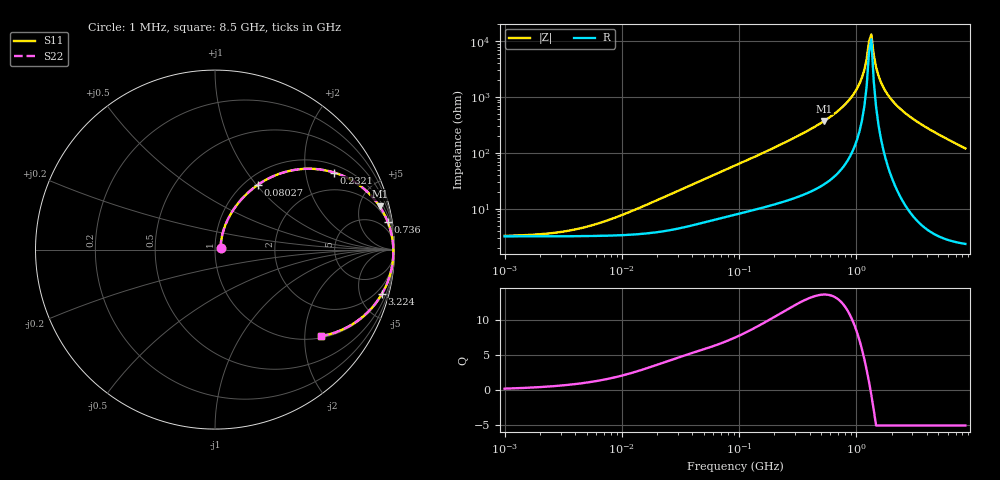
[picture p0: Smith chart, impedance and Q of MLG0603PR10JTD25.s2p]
! S-Parameter Data Generated by TDK Corporation
! Copyright(C) 2025 TDK Corporation.
! All Rights Reserved.
! TDK P/N: MLG0603PR10JTD25 (SMD / SMT Inductor (Coil))
! Property: L=100nH at 300MHz
! Size(LxWxT): 0.6x0.3x0.3mm
! Model Type: s2p (Touchstone File Format Version 1.0)
! Frequency: DC=Yes Start=1MHz Stop=8500MHz 198points Log-sweep
! Model Generated on Feb. 6, 2025
! Terms and conditions regarding TDK Simulation Models:
! 1)This simulation model is being provided solely for informational
!  purposes. Please refer to the specifications of the products in
!  terms of detailed characteristics of such products.
! 2)In no event shall TDK Corporation of any of its subsidiaries be
!  liable for any loss or damage arising, directly or indirectly,
!  from any information contained in this simulation model, including,
!  but not limited to loss or damages arising from any inaccuracies,
!  omissions or errors in connection with such information.
! 3)Any and all copyrights on this simulation model are owned by
!  TDK Corporation.  Duplication or redistribution of this simulation
!  model without prior written permission from TDK Corporation
!  is prohibited.
! 4)This simulation model is subject to any modification or change
!  without any prior notice.
! 5)Neither TDK Corporation nor any of its subsidiaries shall make any
!  warranty, express or implied, including but not limited to the
!  correctness, implied warranties of merchantability and fitness for
!  a particular purpose with respect to this simulation models.
! 6)The use of this simulation model shall be deemed to have consented
!  to the terms and conditions hereof.
! Port Assignments:
!  1 ---@@@--- 2
! Applicable Conditions:
!  Temperature = 25 degC
!  DC Bias Current = 0 A
!  Small Signal Operation
# Hz S MA R 50
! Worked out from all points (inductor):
!   197 points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, 1 MHz to 8.5 GHz, reference 50 ohm
!   read as one part in series: L = 109 nH near 15.95 MHz
!   highest Q = 13.5 at 532.8 MHz (marker M1), where L = 111 nH
!   self-resonance near 1.281 GHz
!   S11 on the Smith chart (normalised r, x): 1 MHz: 1.06, +0.01; 80.27 MHz: 1.15, +1.02; 232.1 MHz: 1.26, +2.88; 736 MHz: 2, +12; 3.224 GHz: 1.13, -7.45; 8.5 GHz: 1.05, -2.41
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1000000  0.03175 11.9  0.969 -0.4  0.969 -0.4  0.03175 11.9
4587603  0.04401 42.8  0.9682 -1.8  0.9682 -1.8  0.04401 42.8
2.10461e7  0.1424 67.1  0.9537 -7.9  0.9537 -7.9  0.1424 67.1
8.027222e7  0.4354 56.4  0.841 -25.5  0.841 -25.5  0.4354 56.4
9.219544e7  0.4805 53.9  0.8154 -28.4  0.8154 -28.4  0.4805 53.9
2.320976e8  0.7899 32.9  0.5459 -51.9  0.5459 -51.9  0.7899 32.9
4.229561e8  0.9194 19.2  0.3301 -66.5  0.3301 -66.5  0.9194 19.2
5.327649e8  0.9487 14.7  0.2539 -71.1  0.2539 -71.1  0.9487 14.7
7.359901e8  0.9753 9.0  0.1568 -76.5  0.1568 -76.5  0.9753 9.0
9.270694e8  0.9863 5.3  0.09311 -78.9  0.09311 -78.9  0.9863 5.3
1.064771e9  0.9905 3.2  0.05647 -78.7  0.05647 -78.7  0.9905 3.2
1.167757e9  0.9923 1.8  0.03256 -75.4  0.03256 -75.4  0.9923 1.8
1.222927e9  0.993 1.1  0.02088 -69.8  0.02088 -69.8  0.993 1.1
1.280704e9  0.9935 0.4  0.0101 -49.4  0.0101 -49.4  0.9935 0.4
1.34121e9  0.9938 -0.2  0.007559 34.4  0.007559 34.4  0.9938 -0.2
1.404574e9  0.9939 -0.9  0.0174 69.1  0.0174 69.1  0.9939 -0.9
1.540426e9  0.9937 -2.3  0.04097 80.0  0.04097 80.0  0.9937 -2.3
1.689417e9  0.9928 -3.7  0.06539 81.8  0.06539 81.8  0.9928 -3.7
1.940355e9  0.9901 -5.9  0.1031 81.5  0.1031 81.5  0.9901 -5.9
3.224109e9  0.9617 -15.0  0.2582 74.1  0.2582 74.1  0.9617 -15.0
5.115526e9  0.8969 -25.4  0.4289 63.7  0.4289 63.7  0.8969 -25.4
8.5e9  0.7618 -39.3  0.6331 49.6  0.6331 49.6  0.7618 -39.3
